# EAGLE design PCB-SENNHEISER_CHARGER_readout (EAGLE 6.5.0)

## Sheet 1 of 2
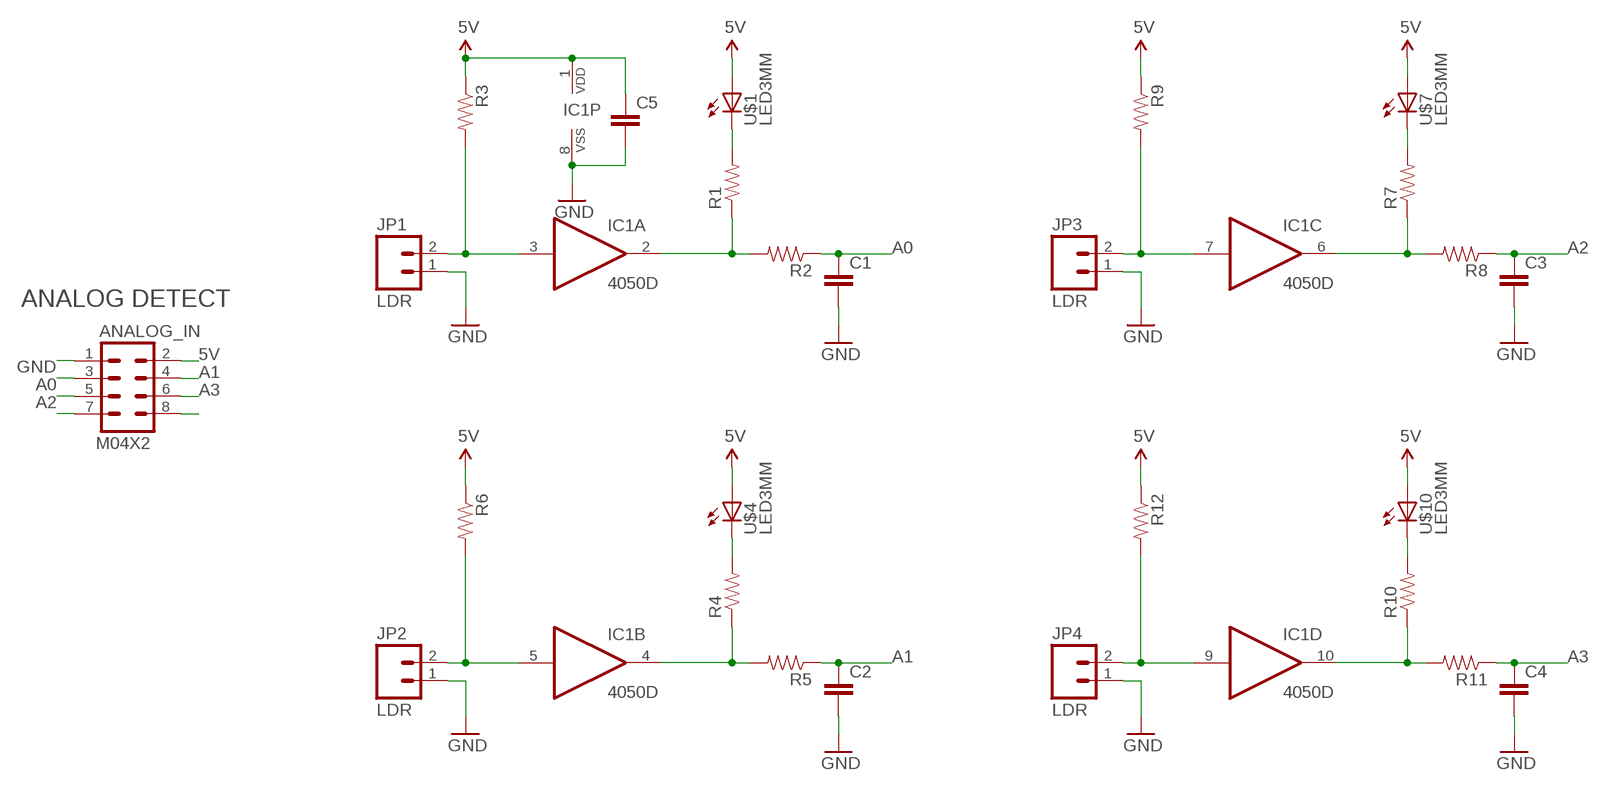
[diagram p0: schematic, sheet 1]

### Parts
ANALOG_IN  M04X2  [2X4]
C1  CAP0603-CAP  [0603-CAP]
C2  CAP0603-CAP  [0603-CAP]
C3  CAP0603-CAP  [0603-CAP]
C4  CAP0603-CAP  [0603-CAP]
C5  CAP0603-CAP  [0603-CAP]
IC1  4050D  [SO16]
JP1  LDR  M02PTH  [1X02]
JP2  LDR  M02PTH  [1X02]
JP3  LDR  M02PTH  [1X02]
JP4  LDR  M02PTH  [1X02]
R1  RESISTOR0603-RES  [0603-RES]
R2  RESISTOR0603-RES  [0603-RES]
R3  RESISTOR0603-RES  [0603-RES]
R4  RESISTOR0603-RES  [0603-RES]
R5  RESISTOR0603-RES  [0603-RES]
R6  RESISTOR0603-RES  [0603-RES]
R7  RESISTOR0603-RES  [0603-RES]
R8  RESISTOR0603-RES  [0603-RES]
R9  RESISTOR0603-RES  [0603-RES]
R10  RESISTOR0603-RES  [0603-RES]
R11  RESISTOR0603-RES  [0603-RES]
R12  RESISTOR0603-RES  [0603-RES]
U$1  LED3MM  [LED3MM]
U$4  LED3MM  [LED3MM]
U$7  LED3MM  [LED3MM]
U$10  LED3MM  [LED3MM]

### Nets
5V [PWR]: ANALOG_IN.2 C5.1 IC1.1(P:VDD) R3.1 R6.1 R9.1 R12.1 U$1.A U$4.A U$7.A U$10.A
A0: ANALOG_IN.3 C1.1 R2.1
A1: ANALOG_IN.4 C2.1 R5.1
A2: ANALOG_IN.5 C3.1 R8.1
A3: ANALOG_IN.6 C4.1 R11.1
GND [PWR]: ANALOG_IN.1 C1.2 C2.2 C3.2 C4.2 C5.2 IC1.8(P:VSS) JP1.1 JP2.1 JP3.1 JP4.1
N$1: IC1.3(A:I) JP1.2 R3.2
N$2: R1.2 U$1.K(C)
N$3: IC1.2(A:O) R1.1 R2.2
N$4: IC1.5(B:I) JP2.2 R6.2
N$5: R4.2 U$4.K(C)
N$6: IC1.4(B:O) R4.1 R5.2
N$7: IC1.7(C:I) JP3.2 R9.2
N$8: R7.2 U$7.K(C)
N$9: IC1.6(C:O) R7.1 R8.2
N$10: IC1.9(D:I) JP4.2 R12.2
N$11: R10.2 U$10.K(C)
N$12: IC1.10(D:O) R10.1 R11.2
N$17: ANALOG_IN.8
N$21: ANALOG_IN.7
Unconnected: IC1.11(E:I) IC1.12(E:O) IC1.14(F:I) IC1.15(F:O)

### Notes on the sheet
- ANALOG DETECT

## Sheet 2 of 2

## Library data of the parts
ANALOG_IN = SparkFun:M04X2
C1-C5 = SparkFun:CAP: Capacitor
IC1 = 40xx:4050: Hex non-inverting BUFFER
JP1-JP4 = SparkFun:M02: Header 2
R1-R12 = SparkFun:RESISTOR: Resistor
U$1 U$4 U$7 U$10 = SKAARHOJ:LED: KINGBRIGHT 20MM BIG LAMP

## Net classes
0 default: width 0.203 mm, drill 0.406 mm, clearance 0.203 mm
1 PWR: width 0.406 mm, drill 0.61 mm, clearance 0.203 mm
2 RELAY LINES: width 0.305 mm, clearance 0.203 mm
3 INput lines: clearance 0.203 mm

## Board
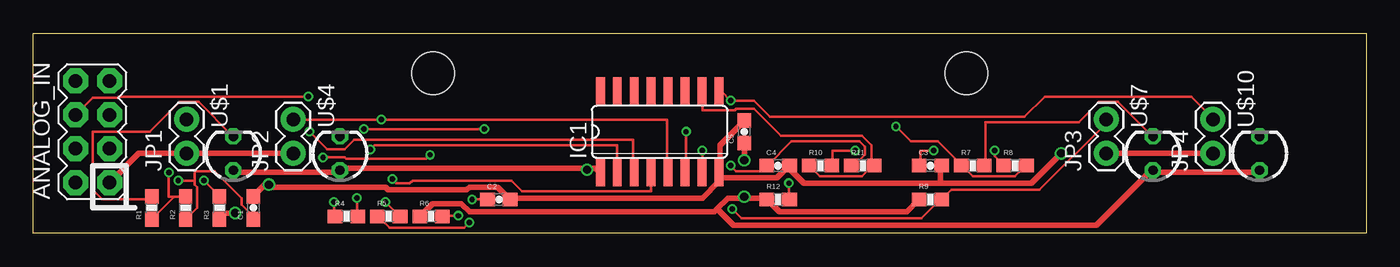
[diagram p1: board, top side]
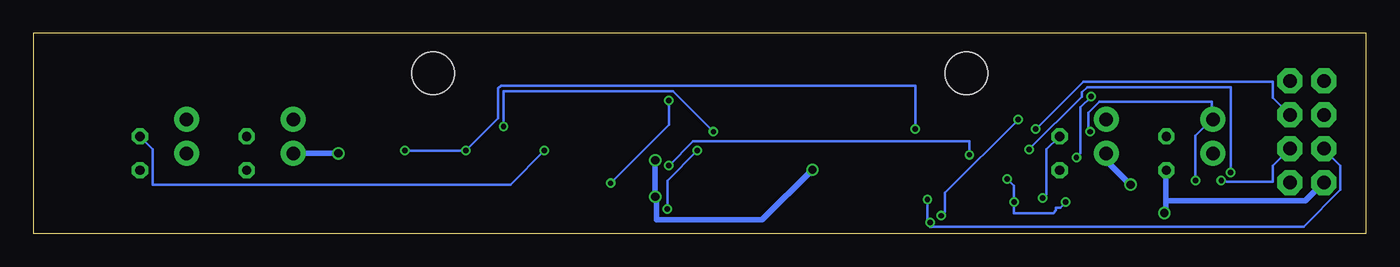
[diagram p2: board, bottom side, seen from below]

Size 100 x 15 mm. Coordinates in mm from the lower left corner, seen from the top.
Outline: 0,0 0,15 100,15 100,0 0,0
Copper layers (1*16): Top 0.035mm / dielectric 1.5mm / Bottom 0.035mm
Design rules "Fusion_eagle_rule_v1.1": minimum track width 6mil, minimum drill 12mil, track to track 6mil, track to pad 6mil, pad to pad 6mil, via to via 6mil, smd to smd 0mil, copper to edge 10mil, drill to drill 10mil, minimum pad ring 10mil, minimum via ring 6mil, stop-mask expansion 2mil, vias tented up to drill 100mil, thermal gap 10mil
Holes 3.2 mm at 30,12 70,12
tRestrict: area 25.4,8.9 to 34.3,15.2; area 65.4,8.9 to 74.3,15.2
bRestrict: area 25.4,8.9 to 33.7,15.2; area 66,8.9 to 74.3,15.2

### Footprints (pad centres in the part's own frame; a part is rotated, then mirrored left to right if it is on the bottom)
2X4 = drill 1.016 pad 1.88 octagon: 1 -3.81,-1.27; 2 -3.81,1.27; 3 -1.27,-1.27; 4 -1.27,1.27; 5 1.27,-1.27; 6 1.27,1.27; 7 3.81,-1.27; 8 3.81,1.27
0603-CAP = smd 1.1 x 1: 1 -0.85,0; 2 0.85,0
SO16 = smd 0.66 x 2.032: 1 -4.445,-3.073; 2 -3.175,-3.073; 3 -1.905,-3.073; 4 -0.635,-3.073; 5 0.635,-3.073; 6 1.905,-3.073; 7 3.175,-3.073; 8 4.445,-3.073; 9 4.445,3.073; 10 3.175,3.073; 11 1.905,3.073; 12 0.635,3.073; 13 -0.635,3.073; 14 -1.905,3.073; 15 -3.175,3.073; 16 -4.445,3.073
1X02 = drill 1.016 pad 1.88: 1 0,0; 2 2.54,0
0603-RES = smd 1.1 x 1: 1 -0.85,0; 2 0.85,0
LED3MM = drill 0.7 pad 1.2 octagon: A -1.27,0; K 1.27,0

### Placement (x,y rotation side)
ANALOG_IN  4.45,7.62 90 top
C1  16.51,1.91 90 top
C2  34.92,2.54 0 top
C3  67.31,5.08 0 top
C4  55.88,5.08 0 top
C5  53.34,7.62 90 top
IC1  46.99,7.62 0 top
JP1  11.5,6 90 top
JP2  19.5,6 90 top
JP3  80.5,6 90 top
JP4  88.5,6 90 top
R1  8.89,1.91 90 top
R2  11.43,1.91 90 top
R3  13.97,1.91 90 top
R4  23.5,1.27 0 top
R5  26.67,1.27 0 top
R6  29.84,1.27 0 top
R7  70.48,5.08 0 top
R8  73.66,5.08 0 top
R9  67.31,2.54 0 top
R10  59.05,5.08 0 top
R11  62.23,5.08 0 top
R12  55.88,2.54 0 top
U$1  15,6 90 top
U$4  23,6 90 top
U$7  84,6 90 top
U$10  92,6 90 top

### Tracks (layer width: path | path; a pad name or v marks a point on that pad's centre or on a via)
5V  (via drill 0.61)
  Top 0.406: v15.14,1.52 14.43,1.52 14.02,1.12 R3.1 | 41.55,4.88 23.16,4.88 23.06,4.78 U$4.A 22.96,4.57 15.14,4.57 15.04,4.67 U$1.A | 41.55,4.88 42.16,4.88 42.47,4.57 IC1.1 | U$10.A 91.95,4.67 91.85,4.57 84.12,4.57 84.02,4.67 U$7.A 83.82,4.67 79.76,0.61 52.53,0.61 51.31,1.83 | 51.31,1.83 52.12,2.64 53.34,2.64 | 51.31,1.83 51.1,1.63 32.72,1.63 32.11,2.23 29.97,2.23 29.06,1.32 R6.1 | 53.34,2.64 54.86,2.64 54.97,2.54 R12.1 55.17,2.44 55.98,1.63 65.53,1.63 66.45,2.54 R9.1 | v53.34,5.49 C5.1 | v53.34,2.74 53.34,2.64 | v41.55,4.78 41.55,4.88
  Bottom 0.406: v15.14,1.52 15.04,1.63 15.04,2.44 | 15.04,2.44 15.04,4.67 U$1.A | 15.04,2.44 4.57,2.44 3.25,3.76 ANALOG_IN.2 | v53.34,5.49 v53.34,2.74 53.24,2.64 53.24,1.02 45.31,1.02 v41.55,4.78
A0  (via drill 0.41)
  Top 0.203: 12.09,3.96 12.09,4.67 13.61,4.67 15.65,2.64 15.65,2.13 16.46,1.32 16.46,1.12 C1.1 | 12.09,3.96 12.09,3.66 12.29,3.45 12.29,1.93 11.48,1.12 R2.1 | v10.87,3.96 12.09,3.96
  Bottom 0.203: v10.87,3.96 10.57,3.96 10.46,3.86 7.01,3.86 7.01,5.08 5.79,6.3 ANALOG_IN.3
A1  (via drill 0.41)
  Top 0.203: v32.72,0.81 32.31,0.41 26.72,0.41 25.91,1.22 R5.1 | C2.1 v32.92,2.54
  Bottom 0.203: v32.92,2.54 32.92,1.02 v32.72,0.81 32.72,0.51 4.67,0.51 1.93,3.25 1.93,5.08 3.15,6.3 ANALOG_IN.4
A2  (via drill 0.41)
  Top 0.203: v67.56,6.2 66.55,6.2 66.55,5.08 C3.1 | v72.14,6.2 72.14,5.79 72.85,5.08 R8.1 | v24.79,7.82 v33.83,7.82
  Bottom 0.203: v72.14,6.2 v67.56,6.2 65.13,8.64 65.13,10.87 64.92,11.07 33.83,11.07 v33.83,7.82 | v24.79,7.82 21.23,11.38 7.01,11.38 7.01,10.16 5.79,8.94 ANALOG_IN.5
A3  (via drill 0.41)
  Top 0.203: R11.1 61.57,5.08 62.38,5.89 62.38,6.5 61.98,6.91 56.9,6.91 55.07,5.08 C4.1 54.97,5.08 54.56,4.67 52.73,4.67 v52.32,5.08 | v29.77,5.89 29.46,5.59 23.47,5.59 23.37,5.69 v21.74,5.69 | v20.62,10.26 6.4,10.26 6.3,10.16 4.47,10.16 3.25,8.94 ANALOG_IN.6
  Bottom 0.203: v52.32,5.08 50.49,6.91 29.77,6.91 v29.77,5.89 | v21.74,5.69 21.44,5.99 21.44,9.45 v20.62,10.26
GND  (via drill 0.61)
  Top 0.406: C1.2 16.56,2.85 17.37,3.66 v17.68,3.66 17.88,3.45 26.42,3.45 26.62,3.25 32.51,3.25 32.72,3.45 34.85,3.45 35.66,2.64 C2.2 35.87,2.54 35.97,2.64 50.19,2.64 51.41,3.86 51.41,4.47 IC1.8 | ANALOG_IN.1 5.79,3.86 7.92,5.99 11.48,5.99 JP1.1 11.68,5.99 19.41,5.99 JP2.1 | JP3.1 80.57,5.99 JP4.1 | C5.2 53.34,8.43 51.51,6.6 51.51,4.67 IC1.8 | IC1.8 51.51,4.17 55.78,4.17 56.69,5.08 C4.2 56.69,4.88 57.81,3.76 68.07,3.76 | 68.07,3.76 68.07,5.08 C3.2 | v77.11,5.99 74.88,3.76 68.07,3.76
  Bottom 0.406: v17.68,3.66 19.41,5.38 19.41,5.99 JP2.1 | v77.11,5.99 80.47,5.99 JP3.1
N$1  (via drill 0.41)
  Top 0.203: v12.8,3.96 13.92,2.85 R3.2 | v20.73,7.62 22.05,6.3 23.37,6.3 24.08,7.01 45.01,7.01 45.01,4.57 IC1.3
  Bottom 0.203: v12.8,3.96 12.8,7.32 11.58,8.53 JP1.2 11.58,8.64 11.58,9.86 20.02,9.86 20.83,9.04 20.83,7.72 v20.73,7.62
N$2
  Top 0.203: R1.2 8.84,2.74 8.64,2.54 5.18,2.54 4.47,3.25 4.47,7.62 8.74,7.62 10.97,9.86 12.39,9.86 14.94,7.32 U$1.K
N$3  (via drill 0.41)
  Top 0.203: 10.52,2.69 10.57,2.74 11.38,2.74 R2.2 | 10.52,2.69 8.94,1.12 R1.1 | v25.3,6.3 25.6,6.6 43.79,6.6 43.79,4.57 IC1.2 | v10.16,4.57 10.16,2.74 10.46,2.74 10.52,2.69
  Bottom 0.203: v25.3,6.3 21.34,10.26 21.34,10.57 20.93,10.97 10.16,10.97 v10.16,4.57
N$4  (via drill 0.41)
  Top 0.203: v31.9,1.32 30.79,1.32 R6.2 | JP2.2 v26.11,8.53 47.55,8.53 47.55,4.57 IC1.5
  Bottom 0.203: v31.9,1.32 31.6,1.63 31.6,3.05 v26.11,8.53
N$5  (via drill 0.41)
  Top 0.203: v24.28,2.64 24.28,1.32 R4.2
  Bottom 0.203: v24.28,2.64 23.98,2.95 23.98,6.3 23.06,7.21 U$4.K
N$6  (via drill 0.41)
  Top 0.203: v22.55,2.34 22.55,1.32 R4.1 | v26.42,2.34 27.43,1.32 R5.2 | v26.92,4.06 27.23,3.76 28.25,3.76 28.45,3.96 35.87,3.96 36.68,3.15 46.33,3.15 46.33,4.47 IC1.4
  Bottom 0.203: v22.55,2.34 22.96,1.93 23.27,1.93 23.27,1.73 23.47,1.52 26.42,1.52 v26.42,2.34 26.42,3.56 v26.92,4.06
N$7  (via drill 0.41)
  Top 0.203: JP3.2 80.47,8.53 80.47,8.23 75.49,3.25 68.89,3.25 68.17,2.54 R9.2 68.07,2.54 66.65,1.12 53.14,1.12 v52.43,1.83 | v50.19,6.2 50.19,4.57 IC1.7
  Bottom 0.203: v50.19,6.2 52.43,3.96 v52.43,1.83
N$8
  Top 0.203: R7.2 71.42,5.08 71.42,8.33 78.44,8.33 79.96,9.86 81.38,9.86 83.92,7.32 U$7.K
N$9  (via drill 0.41)
  Top 0.203: 69.7,5.08 70.51,4.27 73.66,4.27 74.47,5.08 R8.2 | v48.97,7.62 48.97,4.57 IC1.6 | v64.72,8.03 65.84,6.91 67.87,6.91 69.7,5.08 | 69.7,5.08 R7.1
  Bottom 0.203: v48.97,7.62 52.02,10.67 64.72,10.67 v64.72,8.03
N$10  (via drill 0.41)
  Top 0.203: v56.69,3.76 56.69,2.54 R12.2 | IC1.9 51.51,10.67 51.61,10.67 v52.32,9.96 54.05,9.96 55.27,8.74 74.37,8.74 75.89,10.26 86.87,10.26 88.49,8.64 JP4.2
  Bottom 0.203: v56.69,3.76 52.32,8.13 v52.32,9.96
N$11  (via drill 0.41)
  Top 0.203: v61.67,6.2 59.94,6.2 59.94,5.08 R10.2
  Bottom 0.203: v61.67,6.2 64.21,3.66 91.03,3.66 91.03,6.3 91.95,7.21 U$10.K
N$12
  Top 0.203: R10.1 58.22,5.08 59.03,4.27 62.18,4.27 62.99,5.08 R11.2 62.89,5.08 62.89,6.6 62.18,7.32 56.08,7.32 54.05,9.35 52.73,9.35 52.63,9.25 50.19,9.25 50.19,10.67 IC1.10

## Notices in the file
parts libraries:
SparkFun: Licensing: CC v3.0 Share-Alike You are welcome to use this library for commercial purposes.
